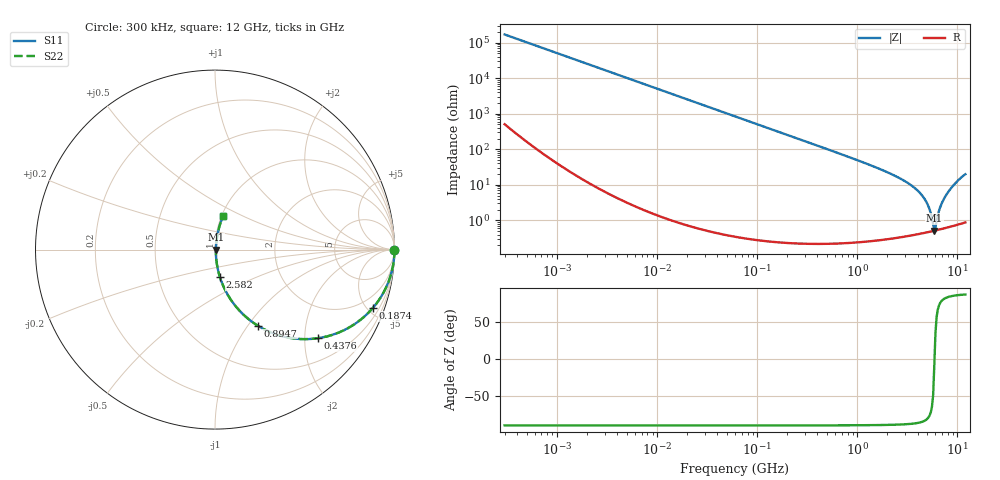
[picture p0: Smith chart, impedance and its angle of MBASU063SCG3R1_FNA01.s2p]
! MBASU063SCG3R1_FNA01  S-PARAMETER MODEL  ( General Type )
! Model Generated by TAIYO YUDEN Corporation (http://www.ty-top.com)
! Version 2.0
! TAIYO YUDEN Control No. 141022
! Copyright(c) 2013 TAIYO YUDEN CO.,LTD. All Rights Reserved.
! Product Description (link to TY-COMPAS)
! https://ds.yuden.co.jp/TYCOMPAS/or/detail?pn=MBASU063SCG3R1CFNA01&u=M
! Products Name : Multilayer Ceramic Capacitors
! Characteristics :
!  Capacitance : 3.1 pF , Rated Voltage : 50V , TCC : CG / C0G
!  Case Size : 0.6 x 0.3 / 0.024 x 0.012 [mm/inch] , Thickness : 0.3 / 0.012 [mm/inch]
!  (Conditions: Temperature = 25 degC , DC Bias Current/Voltage = 0A / 0V)
! External Node Assignments :
!  1  o---| |---o  2
! GND o---------o GND
! Frequency Range : 0.3MHz  -  12000MHz  [ 401 STEP ]
# MHz S RI R 50
! Freq[MHz].  S11 Real  S11 Imag  S21 Real  S21 Imag  S12 Real  S12 Imag  S22 Real  S22 Imag
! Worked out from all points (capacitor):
!   401 points, 300 kHz to 12 GHz, reference 50 ohm
!   read as one part in series: C = 3.13 pF near 316.3 kHz
!   lowest |Z| = 518 mohm at 5.869 GHz (marker M1)
!   series resonance near 5.898 GHz, so ESL is about 230 pH
!   S11 on the Smith chart (normalised r, x): 300 kHz: open; 187.4 MHz: 1.00, -5.43; 437.6 MHz: 1.00, -2.31; 894.7 MHz: 1.00, -1.11; 2.582 GHz: 1.01, -0.32; 12 GHz: 1.02, +0.40
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0.3  1 -0.000589  2.11e-06 0.000589  2.11e-06 0.000589  1 -0.000589
1.769972  1 -0.00348  1.39e-05 0.00348  1.39e-05 0.00348  1 -0.00348
10.44266  0.9996 -0.0205  0.000426 0.0205  0.000426 0.0205  0.9996 -0.0205
60  0.9863 -0.1162  0.0137 0.1162  0.0137 0.1162  0.9863 -0.1162
187.4445  0.8802 -0.3243  0.1198 0.3243  0.1198 0.3243  0.8802 -0.3243
353.9943  0.6723 -0.4686  0.3277 0.4686  0.3277 0.4686  0.6723 -0.4686
437.5599  0.5723 -0.4938  0.4277 0.4938  0.4277 0.4938  0.5723 -0.4938
894.6982  0.2371 -0.4232  0.7629 0.4232  0.7629 0.4232  0.2371 -0.4232
1331.232  0.1182 -0.3193  0.8818 0.3193  0.8818 0.3193  0.1182 -0.3193
2088.533  0.0461 -0.2029  0.9539 0.2029  0.9539 0.2029  0.0461 -0.2029
2581.562  0.0279 -0.1546  0.9721 0.1546  0.9721 0.1546  0.0279 -0.1546
3642.919  0.0112 -0.0853  0.9888 0.0853  0.9888 0.0853  0.0112 -0.0853
4502.883  0.00654 -0.0469  0.9935 0.0469  0.9935 0.0469  0.00654 -0.0469
5140.631  0.00526 -0.0238  0.9947 0.0238  0.9947 0.0238  0.00526 -0.0238
5715.274  0.00504 -0.00572  0.995 0.00572  0.995 0.00572  0.00504 -0.00572
5868.704  0.00509 -0.000808  0.9949 0.000808  0.9949 0.000808  0.00509 -0.000808
6026.253  0.00519 0.0036  0.9948 -0.0036  0.9948 -0.0036  0.00519 0.0036
6188.031  0.00533 0.00799  0.9947 -0.00799  0.9947 -0.00799  0.00533 0.00799
6699.894  0.00604 0.0219  0.994 -0.0219  0.994 -0.0219  0.00604 0.0219
7648.807  0.0085 0.0488  0.9915 -0.0488  0.9915 -0.0488  0.0085 0.0488
9454.42  0.0185 0.1057  0.9815 -0.1057  0.9815 -0.1057  0.0185 0.1057
12000  0.0459 0.1884  0.9541 -0.1884  0.9541 -0.1884  0.0459 0.1884
